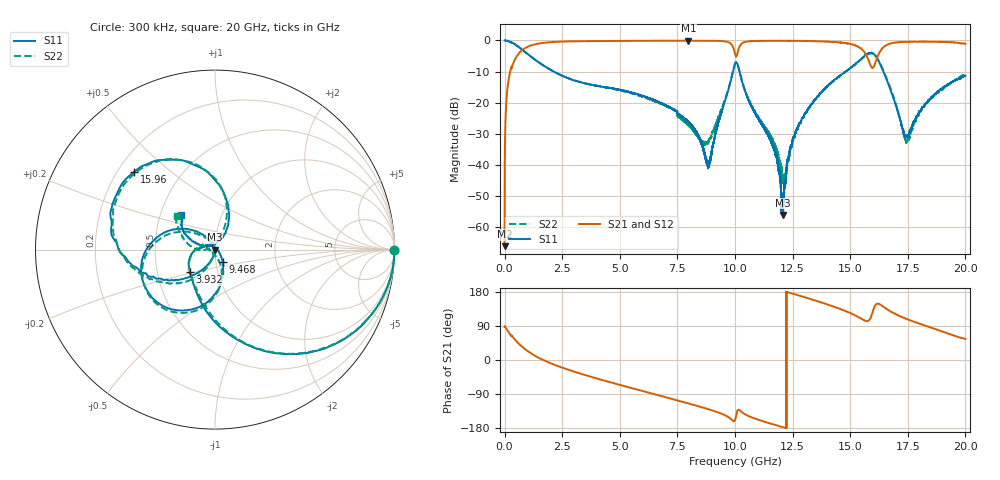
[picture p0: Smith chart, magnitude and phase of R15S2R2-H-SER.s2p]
!{R15S2R2}
!Johanson Technology Inc.
!www.johansontechnology.com
!Test Board Conditions:
!Substrate Type  RO4350B
!Substrate Thickness  20 mil
!Substrate Dk  3.66
!TL Type: GCPW
!TL Trace Width  34 mil
!TL Gap  10 mil
!Electrode orientation  Horizontal
!DUT TOPOLOGY	SERIES
!Mounting Pad LxW  26x52 mil
! Created Sat Feb  6 13:50:11 2021
# hz S ma R 50
! 2 Port Network Data from SP1.SP block
! freq  magS11  angS11  magS21  angS21  magS12  angS12  magS22  angS22
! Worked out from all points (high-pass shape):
!   20001 points, 300 kHz to 20 GHz, reference 50 ohm
!   highest |S21| = -0.07 dB at 7.974 GHz (marker M1); lowest = -66.2 dB at 300 kHz (marker M2)
!   |S21| within 3 dB of the highest: 768.1 MHz to 9.959 GHz (9.191 GHz wide, 171 % of centre); 10.14 GHz to 15.53 GHz (5.386 GHz wide, 42 % of centre)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
!   lowest |S11| = -56.2 dB at 12.08 GHz (marker M3), VSWR 1.00, Z = 49.8 + j0.0218 ohm
!   |S11| at or under -10 dB: 2.133 GHz to 9.912 GHz (7.779 GHz wide, 129 % of centre); 10.19 GHz to 14.81 GHz (4.618 GHz wide, 36.9 % of centre); 16.44 GHz to end of sweep
!   |S22| runs from -45.9 to 0.0 dB; largest |S21 - S12| = 0.014
!   S11 on the Smith chart (normalised r, x): 300 kHz: open; 3.932 GHz: 0.73, -0.19; 9.468 GHz: 1.08, -0.15; 15.96 GHz: 0.27, +0.38; 20 GHz: 0.64, +0.27
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300000  1 -0.2  0.0004888 87.0  0.0003662 96.7  0.9976 -0.1
1.293e8  0.9839 -12.1  0.1747 77.7  0.1756 77.7  0.9831 -12.0
4.693e8  0.8572 -37.3  0.5107 52.4  0.5122 52.5  0.8557 -37.2
1.5193e9  0.4352 -86.0  0.8967 4.6  0.8969 4.5  0.4349 -84.6
3.3343e9  0.2104 -127.6  0.9734 -36.7  0.9731 -36.7  0.2119 -125.3
3.9323e9  0.1883 -137.8  0.9776 -47.6  0.9771 -47.5  0.1892 -136.5
6.6673e9  0.1028 179.2  0.9874 -92.9  0.9883 -92.9  0.1004 174.4
7.9743e9  0.04831 148.5  0.9921 -114.5  0.9907 -114.5  0.04339 171.7
8.8403e9  0.009775 45.3  0.9893 -129.7  0.989 -129.7  0.02325 -114.1
9.4683e9  0.08192 -58.9  0.9739 -142.9  0.9734 -143.0  0.08813 -70.2
1.00003e10  0.4174 -128.5  0.6108 -158.4  0.6112 -158.3  0.4234 -125.6
1.02993e10  0.2238 148.8  0.895 -137.6  0.8965 -137.5  0.2268 154.4
1.16303e10  0.02132 108.4  0.9872 -169.3  0.9868 -169.3  0.02518 110.3
1.20753e10  0.001551 171.9  0.9873 -177.3  0.986 -177.3  0.005203 148.7
1.24713e10  0.02196 -100.6  0.9847 175.7  0.9864 175.7  0.02062 -111.2
1.33343e10  0.09496 -115.1  0.9772 159.8  0.9783 159.9  0.09658 -113.0
1.52223e10  0.4135 -161.6  0.8316 117.5  0.8345 117.4  0.4143 -158.8
1.59613e10  0.6256 136.2  0.3619 124.0  0.3626 123.7  0.6167 136.3
1.66673e10  0.1931 65.9  0.8744 131.0  0.8705 131.7  0.2046 71.0
1.74723e10  0.02873 119.2  0.9507 107.6  0.9518 107.8  0.02431 135.3
1.83333e10  0.1008 161.9  0.9563 89.1  0.9533 88.9  0.09908 180.0
2e10  0.2699 133.7  0.8856 55.5  0.8781 55.3  0.2843 137.8
